PROGRAM MAIN
VAR
	fbEventInfoRecord			:FB_EventInfo;
	fbTon						:TON;
END_VAR

fbTon(IN:=NOT fbTon.Q, PT:=T#1S);
IF fbTon.Q THEN
	fbEventInfoRecord.iID := fbEventInfoRecord.iID + 1;
	fbEventInfoRecord.wsMsg := WCONCAT("中文报警信息测试",TO_WSTRING(fbEventInfoRecord.iID));
	fbEventInfoRecord.M_SendMsg();
	
	fbEventInfoRecord.wsMsg := "同周期内多次调用";		// 准备发送的内容
	fbEventInfoRecord.M_SendMsg();					// 调用即发送,程序中可多次调用
END_IF

fbEventInfoRecord(
	sSourceName:= 'Main', 
	iID:= , 
	wsMsg:= , 
	bInited=> );

END_PROGRAM
